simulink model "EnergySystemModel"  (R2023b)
settings: Solver=VariableStepAuto  StartTime=0.0  StopTime=365  RelTol=1e-3

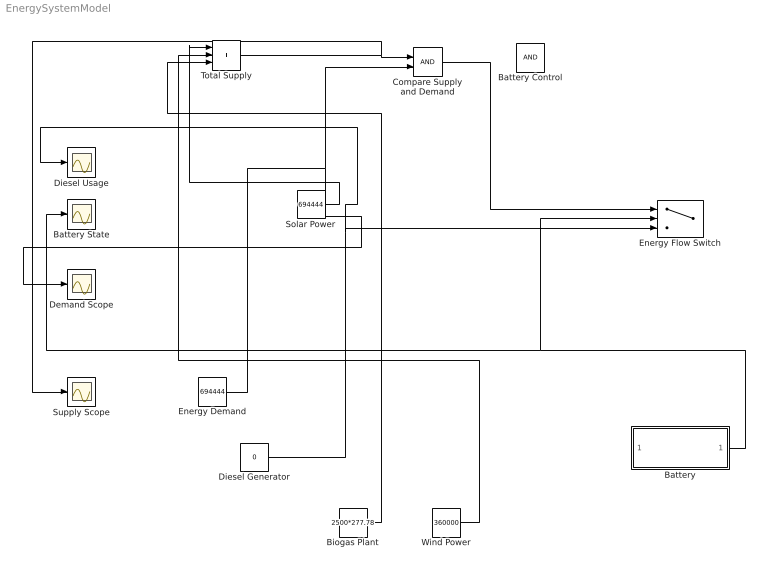
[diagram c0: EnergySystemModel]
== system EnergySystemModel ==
  Battery : Subsystem
  Battery Control : RelationalOperator  OutDataTypeStr=boolean  RndMeth=Simplest
  Battery State : Scope
  Biogas Plant : Constant  Value=2500*277.78
  Compare Supply and Demand : RelationalOperator  OutDataTypeStr=boolean  RndMeth=Simplest
  Demand Scope : Scope
  Diesel Generator : Constant  Value=0
  Diesel Usage : Scope
  Energy Demand : Constant  Value=694444
  Energy Flow Switch : Switch  Criteria=u2 > Threshold
  Solar Power : Constant  Value=694444
  Supply Scope : Scope
  Total Supply : Sum  Inputs=+++
  Wind Power : Constant  Value=360000
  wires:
  Solar Power/1 -> Total Supply/1
  Wind Power/1 -> Total Supply/2
  Biogas Plant/1 -> Total Supply/3
  Total Supply/1 -> Compare Supply and Demand/1, Supply Scope/1
  Energy Demand/1 -> Demand Scope/1, Compare Supply and Demand/2
  Compare Supply and Demand/1 -> Energy Flow Switch/1
  Battery/1(Out1) -> Energy Flow Switch/2, Battery State/1
  Diesel Generator/1 -> Diesel Usage/1, Energy Flow Switch/3

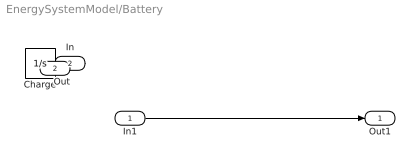
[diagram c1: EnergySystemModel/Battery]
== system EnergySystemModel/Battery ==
  In1 : Inport
  In : Inport  Port=2
  Charge : Integrator
  Out1 : Outport
  Out : Outport  Port=2
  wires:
  In1/1 -> Out1/1
  In/1 -> Charge/1
  Charge/1 -> Out/1
